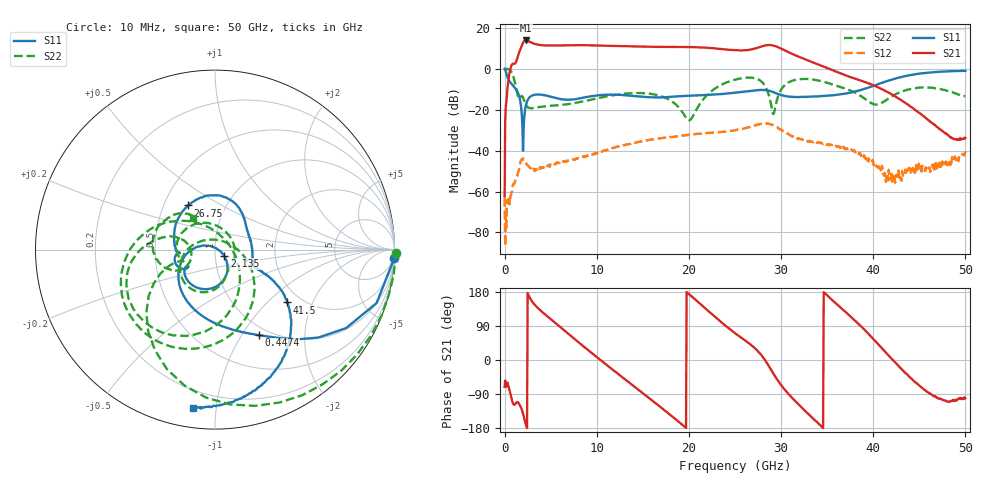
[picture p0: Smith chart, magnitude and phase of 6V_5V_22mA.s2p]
! MARKI MICROWAVE INC.
! Date:  1/07/2020
! Model Number:  APM-6849CH
! Description:  2-port Small Signal S-parameter data for APM-6849CH
! Frequency Range:  10 MHz to 50 GHz
! Port Configuration:  PORT 1: Input
!  PORT 2: Output
! Bias Condition: Vc = +6V, Vb = +5V
! APM-6849CH s2p files are only valid for small signal conditions (below -5 dBm input power)
!S2P File: Measurements: Mag<S11> Ang<S11>, Mag<S21> Ang<S21>, Mag<S12> Ang<S12>, Mag<S22> Ang<S22>!row 1
# Hz S  dB  R 50
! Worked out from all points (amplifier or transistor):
!   801 points, 10 MHz to 50 GHz, reference 50 ohm
!   highest |S21| = 13.8 dB at 2.322 GHz (marker M1)
!   |S21| within 3 dB of that: 1.832 GHz to 15.1 GHz (13.26 GHz wide, 157 % of centre)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
!   unconditionally stable (mu >= 1): 153.3 MHz to end of sweep
!   at 8.321 GHz: K = 18.82, MAG = 11.8 dB, |S12| = -43.5 dB
!   at 25 GHz: K = 3.72, MAG = 10.9 dB, |S12| = -30.0 dB
!   at 50 GHz: K = 498.14, MAG = -26.7 dB, |S12| = -40.5 dB
!   S11 on the Smith chart (normalised r, x): 10 MHz: 0, -42; 447.4 MHz: 0.89, -1.19; 2.135 GHz: 1.11, -0.08; 26.75 GHz: 0.66, +0.36; 41.5 GHz: 1.69, -1.32; 50 GHz: 0.10, -0.87
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1e7  -0.00 -2.7  -62.36 -70.7  -63.21 97.0  0.06 -1.2
4.474125e8  -5.43 -62.9  -4.70 -71.3  -66.06 13.2  -0.35 -51.2
1.5097e9  -12.34 -147.5  6.95 -112.9  -50.08 -66.7  -14.25 -160.9
2.134575e9  -24.22 -33.6  13.54 -153.9  -44.36 -145.5  -15.51 117.1
2.322038e9  -17.80 -57.0  13.81 -170.5  -45.97 -159.7  -17.52 85.0
3.071888e9  -12.93 -102.1  12.48 151.9  -49.35 -168.3  -19.28 10.4
4.571588e9  -13.15 -139.5  11.36 116.8  -47.56 175.1  -18.26 -34.2
8.383325e9  -14.27 -146.4  11.48 39.7  -43.29 136.9  -16.13 -66.6
1.169516e10  -12.65 -163.0  11.16 -24.8  -38.87 102.6  -13.01 -91.2
1.425715e10  -13.42 -173.6  10.89 -73.5  -36.08 67.8  -11.86 -118.6
1.669416e10  -14.03 -174.7  10.70 -119.8  -34.17 32.6  -13.05 -151.5
2.038092e10  -13.12 177.7  10.56 166.4  -32.04 -22.9  -23.65 43.7
2.269296e10  -12.59 166.1  10.01 116.8  -31.19 -62.7  -10.10 -45.2
2.5005e10  -11.69 147.3  9.04 70.9  -30.01 -104.4  -5.33 -94.5
2.675465e10  -10.80 121.5  9.41 39.6  -28.27 -145.0  -4.36 -136.8
2.85043e10  -10.53 78.4  11.51 -9.4  -26.68 152.0  -10.62 148.3
2.981654e10  -12.55 46.3  10.25 -59.9  -29.47 100.6  -11.87 -58.3
3.137872e10  -13.74 22.6  6.92 -104.4  -33.10 66.2  -5.67 -113.2
3.337832e10  -13.62 -3.0  3.18 -152.0  -35.72 31.5  -5.23 -152.1
4.15017e10  -6.07 -36.3  -11.26 16.5  -51.27 151.9  -15.08 -150.1
4.168916e10  -5.76 -37.5  -11.69 11.4  -49.37 127.8  -14.52 -149.8
5e10  -0.98 -97.9  -33.83 -100.9  -40.46 -62.8  -13.44 124.9
